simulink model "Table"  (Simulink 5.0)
settings: Solver=FixedStepDiscrete  SolverMode=SingleTasking  StartTime=0.0  StopTime=inf  FixedStep=samplePeriod  RelTol=1e-3  AbsTol=1e-6
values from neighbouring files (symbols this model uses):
  a0 = zeros(1, nAct)    [initialize.m]    (also in quake.m = 0; rspect.m = 1)
  actParamsX = [bulkModulus	* pressCanon,    [initialize.m]
  actParamsY = [bulkModulus	* pressCanon,    [initialize.m]
  actParamsZ = [bulkModulus	* pressCanon,    [initialize.m]
  azMask = zeros(nAcc, 1)    [initialize.m]
  bal = [[ 1  1  1  1  0  0  0  0  0  0  0  0]    [initialize.m]
  cmap = jet    [initialize.m]    (also in tableAnimation.m = self.cmap)
  ea_t = zeros(3, nAcc)    [initialize.m]
  faces = nAct               			+ [ 1  2  3  4    [initialize.m]    (also in tableAnimation.m = self.faces)
  flowCanon = 63090.2    [initialize.m]
  fmax = zeros(nAct, 1)    [initialize.m]
  gasConstant = 1.8    [initialize.m]
  gee = 1.0    (= 1)    [initialize.m]    (also in accelA2T.m = h(24); accelT2A.m = h(24); Test.m)
  inertia = [Ixx 0 0; 0 Iyy 0; 0 0 Izz]    [initialize.m]
  inertiaCanon = 0.1130    (= 0.113)    [initialize.m]
  linAccelCanon = 9800.0    (= 9800)    [initialize.m]    (also in accelA2T.m = h(19); accelT2A.m = h(19); Test.m)
  lines = nAct               			+ [ 1  2  3  4  1    				5  6  7  8  5    				9 10 11 12  9    				0  2  6 10       				0  3  7 11       				0  4  8 12  0];  	lines(find(lines==nAct)) = 0    [initialize.m]    (also in tableAnimation.m = self.lines; viewer.m = 1)
  linVelocCanon = 1000.0    (= 1000)    [initialize.m]    (also in Test.m)
  mass = [massX massY massZ]'    [initialize.m]
  massCanon = 0.4535924e-06    (= 4.535924e-07)    [initialize.m]
  maxDispl = [maxDisplX  			maxDisplY  			maxDisplZ  			maxDisplZ * linVelocCanon / rollRadius  * 180/pi  			maxDisplZ * linVelocCanon / pitchRadius * 180/pi  			min(maxDisplX, maxDisplY) * linVelocCanon / yawRadius * 180/pi]    [initialize.m]
  maxOilVolume = volume * (1 - (precharge/supplyPress)^(1/gasConstant))    (= 32.2704137442)    [initialize.m]
  maxVeloc = [maxVelocX  			maxVelocY  			maxVelocZ  			maxVelocZ * linVelocCanon / rollRadius  * 180/pi  			maxVelocZ * linVelocCanon / pitchRadius * 180/pi  			min(maxVelocX, maxVelocY) * linVelocCanon / yawRadius * 180/pi]    [initialize.m]
  minDispl = -maxDispl    [initialize.m]
  minVeloc = -maxVeloc    [initialize.m]
  nAct = size(rt_t, 2)    [initialize.m]    (also in tableAnimation.m = self.nAct)
  precharge = 2000    [initialize.m]
  pumpFlow = 1e10    (= 10000000000)    [initialize.m]
  ra_t = [  -20.0   -20.0   -92.0 -2590.0  2590.0   -62.0 -2133.0 -2133.0  2133.0  2133.0   -62.0    [initialize.m]    (also in accelA2T.m = [-h9   -h9 -h15 -h10  h10 -h14 -h12 -h12  h12  h12 -h16; accelT2A.m = [-h9   -h9 -h15 -h10  h10 -h14 -h12 -h12  h12  h12 -h16)
  rb_w = [-5692.1 -5692.1  5692.1  5692.1 -2500.0 -2500.0  2500.0  2500.0 -2400.0 -2400.0  2400.0  2400.0    [initialize.m]    (also in tableAnimation.m = rtxrb_w(:,end-nAct+1:end); positT2A.m = [-h4 -h4  h4  h4 -h1 -h1  h1  h1 -h6 -h6  h6  h6)
  returnPress = 50    [initialize.m]
  rgt = -rtg    [initialize.m]
  rotAccelCanon = 1    [initialize.m]    (also in accelA2T.m = h(22); accelT2A.m = h(22); Test.m)
  rotForceCanon = 1000    [initialize.m]    (also in forceA2T.m = h(23); Test.m)
  rotVelocCanon = 1    [initialize.m]    (also in accelA2T.m = h(21); accelT2A.m = h(21); Test.m)
  rt_t = [-3106.4 -3106.4  3106.4  3106.4 -2500.0 -2500.0  2500.0  2500.0 -2400.0 -2400.0  2400.0  2400.0    [initialize.m]    (also in positT2A.m = [rt_tx rt_ty rt_tz])
  rtg = cg    [initialize.m]
  rtx_t = [rt_t	topPlane.topLeft(:)  topPlane.topRight(:)  					topPlane.botRight(:) topPlane.botLeft(:)   					midPlane.topLeft(:)  midPlane.topRight(:)  					midPlane.botRight(:) midPlane.botLeft(:)   					botPlane.topLeft(:)  botPlane.topRight(:)  					botPlane.botRight(:) botPlane.botLeft(:)]    [initialize.m]
  samplePeriod = 1/1024    (= 0.0009765625)    [initialize.m]    (also in viewer.m = eval(getHeaderValue(header, 'DELTA_T')))
  supplyPress = 3000    [initialize.m]
  volume = 160    [initialize.m]    (also in quake.m = volume / 231.0)
  volumeCanon = 3785412.0    (= 3785412)    [initialize.m]
  zlim = [min(rb_w(3,:)) 2*halfLengthZ*lengthCanon]    [initialize.m]
undefined symbols (not defined in the file or in its folder): magnitude
libraries: aerospace x51, simulink x22, simulink_extras x1
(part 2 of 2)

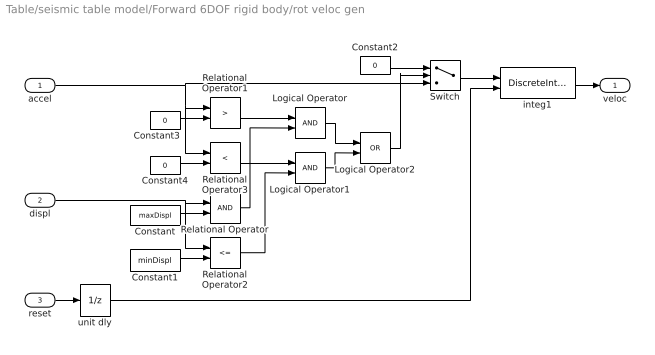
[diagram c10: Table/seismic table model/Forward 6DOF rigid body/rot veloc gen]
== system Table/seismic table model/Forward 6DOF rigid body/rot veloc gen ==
  accel : Inport
  displ : Inport  Port=2
  reset : Inport  Port=3
  Constant : Constant  Value=maxDispl
  Constant1 : Constant  Value=minDispl
  Constant2 : Constant  Value=0
  Constant3 : Constant  Value=0
  Constant4 : Constant  Value=0
  Logical Operator : Logic
  Logical Operator1 : Logic
  Logical Operator2 : Logic  Operator=OR
  Relational Operator : RelationalOperator
  Relational Operator1 : RelationalOperator  Operator=>
  Relational Operator2 : RelationalOperator  Operator=<=
  Relational Operator3 : RelationalOperator  Operator=<
  Switch : Switch  Threshold=0.5
  integ1 : DiscreteIntegrator  ExternalReset=either  LimitOutput=on  UpperSaturationLimit=maxVeloc  LowerSaturationLimit=minVeloc  SampleTime=-1
  unit dly : UnitDelay  SampleTime=-1
  veloc : Outport
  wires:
  reset/1 -> unit dly/1
  displ/1 -> Relational Operator2/1, Relational Operator/1
  Logical Operator1/1 -> Logical Operator2/2
  unit dly/1 -> integ1/2
  Switch/1 -> integ1/1
  Logical Operator2/1 -> Switch/2
  Constant2/1 -> Switch/1
  Logical Operator/1 -> Logical Operator2/1
  Relational Operator3/1 -> Logical Operator1/1
  Constant4/1 -> Relational Operator3/2
  Relational Operator1/1 -> Logical Operator/1
  Constant3/1 -> Relational Operator1/2
  accel/1 -> Switch/3, Relational Operator1/1, Relational Operator3/1
  Constant1/1 -> Relational Operator2/2
  Relational Operator2/1 -> Logical Operator1/2
  Relational Operator/1 -> Logical Operator/2
  Constant/1 -> Relational Operator/2
  integ1/1 -> veloc/1

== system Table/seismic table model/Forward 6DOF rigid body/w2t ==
  rpw : Inport
  11 : Fcn  Expr=cos(u[3])*cos(u[2])-sin(u[3])*sin(u[1])*sin(u[2])
  12 : Fcn  Expr=sin(u[3])*cos(u[2])+cos(u[3])*sin(u[1])*sin(u[2])
  13 : Fcn  Expr=-cos(u[1])*sin(u[2])
  21 : Fcn  Expr=-sin(u[3])*cos(u[1])
  22 : Fcn  Expr=cos(u[3])*cos(u[1])
  23 : Fcn
  31 : Fcn  Expr=cos(u[3])*sin(u[2])+sin(u[3])*sin(u[1])*cos(u[2])
  32 : Fcn  Expr=sin(u[3])*sin(u[2])-cos(u[3])*sin(u[1])*cos(u[2])
  33 : Fcn  Expr=cos(u[1])*cos(u[2])
  9x1->3x3 : simulink/Math Operations/Reshape  OutputDimensionality=Customize  OutputDimensions=[3,3]
  Mux2 : Mux  Orientation=down  Inputs=9
  DCM : Outport
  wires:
  9x1->3x3/1 -> DCM/1
  11/1 -> Mux2/1
  21/1 -> Mux2/2
  31/1 -> Mux2/3
  rpw/1 -> 31/1, 21/1, 11/1, 32/1, 22/1, 12/1, 33/1, 23/1, 13/1
  12/1 -> Mux2/4
  22/1 -> Mux2/5
  32/1 -> Mux2/6
  Mux2/1 -> 9x1->3x3/1
  13/1 -> Mux2/7
  23/1 -> Mux2/8
  33/1 -> Mux2/9

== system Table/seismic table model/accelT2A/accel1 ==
  linacc : Inport
  rotacc : Inport  Port=2
  rotvel : Inport  Port=3
  Sum : Sum  Inputs=+++
  crossprod1 : aerospace/Axes Transformations/3x3 cross product
  crossprod2 : aerospace/Axes Transformations/3x3 cross product
  crossprod3 : aerospace/Axes Transformations/3x3 cross product
  dotprod : simulink/Math Operations/Dot Product
  orient : Constant  Value=ea_t(:,id)
  ra_t : Constant  Value=ra_t(:,id)
  out : Outport
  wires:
  orient/1 -> dotprod/2
  dotprod/1 -> out/1
  linacc/1 -> Sum/1
  Sum/1 -> dotprod/1
  rotacc/1 -> crossprod1/1
  ra_t/1 -> crossprod1/2, crossprod2/2
  crossprod1/1 -> Sum/2
  rotvel/1 -> crossprod2/1, crossprod3/1
  crossprod3/1 -> Sum/3
  crossprod2/1 -> crossprod3/2

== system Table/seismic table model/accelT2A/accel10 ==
  linacc : Inport
  rotacc : Inport  Port=2
  rotvel : Inport  Port=3
  Sum : Sum  Inputs=+++
  crossprod1 : aerospace/Axes Transformations/3x3 cross product
  crossprod2 : aerospace/Axes Transformations/3x3 cross product
  crossprod3 : aerospace/Axes Transformations/3x3 cross product
  dotprod : simulink/Math Operations/Dot Product
  orient : Constant  Value=ea_t(:,id)
  ra_t : Constant  Value=ra_t(:,id)
  out : Outport
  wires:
  crossprod2/1 -> crossprod3/2
  crossprod3/1 -> Sum/3
  rotvel/1 -> crossprod3/1, crossprod2/1
  crossprod1/1 -> Sum/2
  ra_t/1 -> crossprod2/2, crossprod1/2
  rotacc/1 -> crossprod1/1
  Sum/1 -> dotprod/1
  linacc/1 -> Sum/1
  dotprod/1 -> out/1
  orient/1 -> dotprod/2

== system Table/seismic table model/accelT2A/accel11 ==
  linacc : Inport
  rotacc : Inport  Port=2
  rotvel : Inport  Port=3
  Sum : Sum  Inputs=+++
  crossprod1 : aerospace/Axes Transformations/3x3 cross product
  crossprod2 : aerospace/Axes Transformations/3x3 cross product
  crossprod3 : aerospace/Axes Transformations/3x3 cross product
  dotprod : simulink/Math Operations/Dot Product
  orient : Constant  Value=ea_t(:,id)
  ra_t : Constant  Value=ra_t(:,id)
  out : Outport
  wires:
  orient/1 -> dotprod/2
  dotprod/1 -> out/1
  linacc/1 -> Sum/1
  Sum/1 -> dotprod/1
  rotacc/1 -> crossprod1/1
  ra_t/1 -> crossprod1/2, crossprod2/2
  crossprod1/1 -> Sum/2
  rotvel/1 -> crossprod2/1, crossprod3/1
  crossprod3/1 -> Sum/3
  crossprod2/1 -> crossprod3/2

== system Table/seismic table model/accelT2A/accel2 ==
  linacc : Inport
  rotacc : Inport  Port=2
  rotvel : Inport  Port=3
  Sum : Sum  Inputs=+++
  crossprod1 : aerospace/Axes Transformations/3x3 cross product
  crossprod2 : aerospace/Axes Transformations/3x3 cross product
  crossprod3 : aerospace/Axes Transformations/3x3 cross product
  dotprod : simulink/Math Operations/Dot Product
  orient : Constant  Value=ea_t(:,id)
  ra_t : Constant  Value=ra_t(:,id)
  out : Outport
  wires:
  crossprod2/1 -> crossprod3/2
  crossprod3/1 -> Sum/3
  rotvel/1 -> crossprod3/1, crossprod2/1
  crossprod1/1 -> Sum/2
  ra_t/1 -> crossprod2/2, crossprod1/2
  rotacc/1 -> crossprod1/1
  Sum/1 -> dotprod/1
  linacc/1 -> Sum/1
  dotprod/1 -> out/1
  orient/1 -> dotprod/2

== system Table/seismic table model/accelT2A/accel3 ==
  linacc : Inport
  rotacc : Inport  Port=2
  rotvel : Inport  Port=3
  Sum : Sum  Inputs=+++
  crossprod1 : aerospace/Axes Transformations/3x3 cross product
  crossprod2 : aerospace/Axes Transformations/3x3 cross product
  crossprod3 : aerospace/Axes Transformations/3x3 cross product
  dotprod : simulink/Math Operations/Dot Product
  orient : Constant  Value=ea_t(:,id)
  ra_t : Constant  Value=ra_t(:,id)
  out : Outport
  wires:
  orient/1 -> dotprod/2
  dotprod/1 -> out/1
  linacc/1 -> Sum/1
  Sum/1 -> dotprod/1
  rotacc/1 -> crossprod1/1
  ra_t/1 -> crossprod1/2, crossprod2/2
  crossprod1/1 -> Sum/2
  rotvel/1 -> crossprod2/1, crossprod3/1
  crossprod3/1 -> Sum/3
  crossprod2/1 -> crossprod3/2

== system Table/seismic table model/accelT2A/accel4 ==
  linacc : Inport
  rotacc : Inport  Port=2
  rotvel : Inport  Port=3
  Sum : Sum  Inputs=+++
  crossprod1 : aerospace/Axes Transformations/3x3 cross product
  crossprod2 : aerospace/Axes Transformations/3x3 cross product
  crossprod3 : aerospace/Axes Transformations/3x3 cross product
  dotprod : simulink/Math Operations/Dot Product
  orient : Constant  Value=ea_t(:,id)
  ra_t : Constant  Value=ra_t(:,id)
  out : Outport
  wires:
  crossprod2/1 -> crossprod3/2
  crossprod3/1 -> Sum/3
  rotvel/1 -> crossprod3/1, crossprod2/1
  crossprod1/1 -> Sum/2
  ra_t/1 -> crossprod2/2, crossprod1/2
  rotacc/1 -> crossprod1/1
  Sum/1 -> dotprod/1
  linacc/1 -> Sum/1
  dotprod/1 -> out/1
  orient/1 -> dotprod/2

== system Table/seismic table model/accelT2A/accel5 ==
  linacc : Inport
  rotacc : Inport  Port=2
  rotvel : Inport  Port=3
  Sum : Sum  Inputs=+++
  crossprod1 : aerospace/Axes Transformations/3x3 cross product
  crossprod2 : aerospace/Axes Transformations/3x3 cross product
  crossprod3 : aerospace/Axes Transformations/3x3 cross product
  dotprod : simulink/Math Operations/Dot Product
  orient : Constant  Value=ea_t(:,id)
  ra_t : Constant  Value=ra_t(:,id)
  out : Outport
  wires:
  orient/1 -> dotprod/2
  dotprod/1 -> out/1
  linacc/1 -> Sum/1
  Sum/1 -> dotprod/1
  rotacc/1 -> crossprod1/1
  ra_t/1 -> crossprod1/2, crossprod2/2
  crossprod1/1 -> Sum/2
  rotvel/1 -> crossprod2/1, crossprod3/1
  crossprod3/1 -> Sum/3
  crossprod2/1 -> crossprod3/2

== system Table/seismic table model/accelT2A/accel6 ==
  linacc : Inport
  rotacc : Inport  Port=2
  rotvel : Inport  Port=3
  Sum : Sum  Inputs=+++
  crossprod1 : aerospace/Axes Transformations/3x3 cross product
  crossprod2 : aerospace/Axes Transformations/3x3 cross product
  crossprod3 : aerospace/Axes Transformations/3x3 cross product
  dotprod : simulink/Math Operations/Dot Product
  orient : Constant  Value=ea_t(:,id)
  ra_t : Constant  Value=ra_t(:,id)
  out : Outport
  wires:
  crossprod2/1 -> crossprod3/2
  crossprod3/1 -> Sum/3
  rotvel/1 -> crossprod3/1, crossprod2/1
  crossprod1/1 -> Sum/2
  ra_t/1 -> crossprod2/2, crossprod1/2
  rotacc/1 -> crossprod1/1
  Sum/1 -> dotprod/1
  linacc/1 -> Sum/1
  dotprod/1 -> out/1
  orient/1 -> dotprod/2

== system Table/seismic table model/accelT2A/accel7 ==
  linacc : Inport
  rotacc : Inport  Port=2
  rotvel : Inport  Port=3
  Sum : Sum  Inputs=+++
  crossprod1 : aerospace/Axes Transformations/3x3 cross product
  crossprod2 : aerospace/Axes Transformations/3x3 cross product
  crossprod3 : aerospace/Axes Transformations/3x3 cross product
  dotprod : simulink/Math Operations/Dot Product
  orient : Constant  Value=ea_t(:,id)
  ra_t : Constant  Value=ra_t(:,id)
  out : Outport
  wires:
  orient/1 -> dotprod/2
  dotprod/1 -> out/1
  linacc/1 -> Sum/1
  Sum/1 -> dotprod/1
  rotacc/1 -> crossprod1/1
  ra_t/1 -> crossprod1/2, crossprod2/2
  crossprod1/1 -> Sum/2
  rotvel/1 -> crossprod2/1, crossprod3/1
  crossprod3/1 -> Sum/3
  crossprod2/1 -> crossprod3/2

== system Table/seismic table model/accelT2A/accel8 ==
  linacc : Inport
  rotacc : Inport  Port=2
  rotvel : Inport  Port=3
  Sum : Sum  Inputs=+++
  crossprod1 : aerospace/Axes Transformations/3x3 cross product
  crossprod2 : aerospace/Axes Transformations/3x3 cross product
  crossprod3 : aerospace/Axes Transformations/3x3 cross product
  dotprod : simulink/Math Operations/Dot Product
  orient : Constant  Value=ea_t(:,id)
  ra_t : Constant  Value=ra_t(:,id)
  out : Outport
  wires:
  crossprod2/1 -> crossprod3/2
  crossprod3/1 -> Sum/3
  rotvel/1 -> crossprod3/1, crossprod2/1
  crossprod1/1 -> Sum/2
  ra_t/1 -> crossprod2/2, crossprod1/2
  rotacc/1 -> crossprod1/1
  Sum/1 -> dotprod/1
  linacc/1 -> Sum/1
  dotprod/1 -> out/1
  orient/1 -> dotprod/2

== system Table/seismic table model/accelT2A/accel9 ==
  linacc : Inport
  rotacc : Inport  Port=2
  rotvel : Inport  Port=3
  Sum : Sum  Inputs=+++
  crossprod1 : aerospace/Axes Transformations/3x3 cross product
  crossprod2 : aerospace/Axes Transformations/3x3 cross product
  crossprod3 : aerospace/Axes Transformations/3x3 cross product
  dotprod : simulink/Math Operations/Dot Product
  orient : Constant  Value=ea_t(:,id)
  ra_t : Constant  Value=ra_t(:,id)
  out : Outport
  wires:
  orient/1 -> dotprod/2
  dotprod/1 -> out/1
  linacc/1 -> Sum/1
  Sum/1 -> dotprod/1
  rotacc/1 -> crossprod1/1
  ra_t/1 -> crossprod1/2, crossprod2/2
  crossprod1/1 -> Sum/2
  rotvel/1 -> crossprod2/1, crossprod3/1
  crossprod3/1 -> Sum/3
  crossprod2/1 -> crossprod3/2

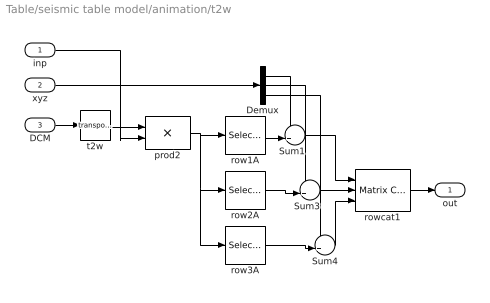
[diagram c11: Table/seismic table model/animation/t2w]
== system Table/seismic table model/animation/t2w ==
  inp : Inport
  xyz : Inport  Port=2
  DCM : Inport  Port=3
  Demux : Demux  Outputs=3
  Sum1 : Sum  Inputs=++|
  Sum3 : Sum  Inputs=++|
  Sum4 : Sum  Inputs=++|
  prod2 : Product  Multiplication=Matrix(*)
  row1A : Selector  InputType=Matrix  Elements=[1 3]  Columns=-1  InputPortWidth=3
  row2A : Selector  InputType=Matrix  Elements=[1 3]  Rows=2  Columns=-1  InputPortWidth=3
  row3A : Selector  InputType=Matrix  Elements=[1 3]  Rows=3  Columns=-1  InputPortWidth=3
  rowcat1 : simulink/Math Operations/Matrix Concatenation  numInports=3  catMethod=Vertical
  t2w : Math  Operator=transpose
  out : Outport
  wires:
  t2w/1 -> prod2/1
  Sum4/1 -> rowcat1/3
  Sum1/1 -> rowcat1/1
  Sum3/1 -> rowcat1/2
  Demux/3 -> Sum4/1
  Demux/2 -> Sum3/1
  row3A/1 -> Sum4/2
  row2A/1 -> Sum3/2
  Demux/1 -> Sum1/1
  prod2/1 -> row2A/1, row3A/1, row1A/1
  DCM/1 -> t2w/1
  inp/1 -> prod2/2
  rowcat1/1 -> out/1
  row1A/1 -> Sum1/2
  xyz/1 -> Demux/1

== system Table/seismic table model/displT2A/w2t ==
  inp : Inport
  xyz : Inport  Port=2
  DCM : Inport  Port=3
  Demux : Demux  Outputs=3
  Sum5 : Sum  Inputs=-+|
  Sum6 : Sum  Inputs=-+|
  Sum7 : Sum  Inputs=-+|
  prod : Product  Multiplication=Matrix(*)
  row1A : Selector  InputType=Matrix  Elements=[1 3]  Columns=-1  InputPortWidth=3
  row2A : Selector  InputType=Matrix  Elements=[1 3]  Rows=2  Columns=-1  InputPortWidth=3
  row3A : Selector  InputType=Matrix  Elements=[1 3]  Rows=3  Columns=-1  InputPortWidth=3
  rowcat : simulink/Math Operations/Matrix Concatenation  numInports=3  catMethod=Vertical
  out : Outport
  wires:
  DCM/1 -> prod/1
  prod/1 -> out/1
  rowcat/1 -> prod/2
  inp/1 -> row3A/1, row2A/1, row1A/1
  xyz/1 -> Demux/1
  row1A/1 -> Sum5/2
  Demux/1 -> Sum5/1
  row2A/1 -> Sum6/2
  row3A/1 -> Sum7/2
  Demux/2 -> Sum6/1
  Demux/3 -> Sum7/1
  Sum6/1 -> rowcat/2
  Sum5/1 -> rowcat/1
  Sum7/1 -> rowcat/3

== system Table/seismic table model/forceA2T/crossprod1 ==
  A : Inport
  B : Inport  Port=2
  colA : Selector  InputType=Matrix  Elements=[1 3]  Rows=-1  Columns=id  InputPortWidth=3
  colB : Selector  InputType=Matrix  Elements=[1 3]  Rows=-1  Columns=id  InputPortWidth=3
  crossprod : aerospace/Axes Transformations/3x3 cross product
  AxB : Outport
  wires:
  colA/1 -> crossprod/1
  colB/1 -> crossprod/2
  A/1 -> colA/1
  B/1 -> colB/1
  crossprod/1 -> AxB/1

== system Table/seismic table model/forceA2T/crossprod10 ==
  A : Inport
  B : Inport  Port=2
  colA : Selector  InputType=Matrix  Elements=[1 3]  Rows=-1  Columns=id  InputPortWidth=3
  colB : Selector  InputType=Matrix  Elements=[1 3]  Rows=-1  Columns=id  InputPortWidth=3
  crossprod : aerospace/Axes Transformations/3x3 cross product
  AxB : Outport
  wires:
  colA/1 -> crossprod/1
  colB/1 -> crossprod/2
  A/1 -> colA/1
  B/1 -> colB/1
  crossprod/1 -> AxB/1

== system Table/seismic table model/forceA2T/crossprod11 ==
  A : Inport
  B : Inport  Port=2
  colA : Selector  InputType=Matrix  Elements=[1 3]  Rows=-1  Columns=id  InputPortWidth=3
  colB : Selector  InputType=Matrix  Elements=[1 3]  Rows=-1  Columns=id  InputPortWidth=3
  crossprod : aerospace/Axes Transformations/3x3 cross product
  AxB : Outport
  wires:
  crossprod/1 -> AxB/1
  B/1 -> colB/1
  A/1 -> colA/1
  colB/1 -> crossprod/2
  colA/1 -> crossprod/1

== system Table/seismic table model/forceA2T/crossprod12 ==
  A : Inport
  B : Inport  Port=2
  colA : Selector  InputType=Matrix  Elements=[1 3]  Rows=-1  Columns=id  InputPortWidth=3
  colB : Selector  InputType=Matrix  Elements=[1 3]  Rows=-1  Columns=id  InputPortWidth=3
  crossprod : aerospace/Axes Transformations/3x3 cross product
  AxB : Outport
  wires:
  colA/1 -> crossprod/1
  colB/1 -> crossprod/2
  A/1 -> colA/1
  B/1 -> colB/1
  crossprod/1 -> AxB/1

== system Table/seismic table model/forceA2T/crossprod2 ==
  A : Inport
  B : Inport  Port=2
  colA : Selector  InputType=Matrix  Elements=[1 3]  Rows=-1  Columns=id  InputPortWidth=3
  colB : Selector  InputType=Matrix  Elements=[1 3]  Rows=-1  Columns=id  InputPortWidth=3
  crossprod : aerospace/Axes Transformations/3x3 cross product
  AxB : Outport
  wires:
  crossprod/1 -> AxB/1
  B/1 -> colB/1
  A/1 -> colA/1
  colB/1 -> crossprod/2
  colA/1 -> crossprod/1

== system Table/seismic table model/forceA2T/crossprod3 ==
  A : Inport
  B : Inport  Port=2
  colA : Selector  InputType=Matrix  Elements=[1 3]  Rows=-1  Columns=id  InputPortWidth=3
  colB : Selector  InputType=Matrix  Elements=[1 3]  Rows=-1  Columns=id  InputPortWidth=3
  crossprod : aerospace/Axes Transformations/3x3 cross product
  AxB : Outport
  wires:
  colA/1 -> crossprod/1
  colB/1 -> crossprod/2
  A/1 -> colA/1
  B/1 -> colB/1
  crossprod/1 -> AxB/1

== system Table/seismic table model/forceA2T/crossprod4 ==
  A : Inport
  B : Inport  Port=2
  colA : Selector  InputType=Matrix  Elements=[1 3]  Rows=-1  Columns=id  InputPortWidth=3
  colB : Selector  InputType=Matrix  Elements=[1 3]  Rows=-1  Columns=id  InputPortWidth=3
  crossprod : aerospace/Axes Transformations/3x3 cross product
  AxB : Outport
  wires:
  crossprod/1 -> AxB/1
  B/1 -> colB/1
  A/1 -> colA/1
  colB/1 -> crossprod/2
  colA/1 -> crossprod/1

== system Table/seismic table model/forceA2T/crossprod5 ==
  A : Inport
  B : Inport  Port=2
  colA : Selector  InputType=Matrix  Elements=[1 3]  Rows=-1  Columns=id  InputPortWidth=3
  colB : Selector  InputType=Matrix  Elements=[1 3]  Rows=-1  Columns=id  InputPortWidth=3
  crossprod : aerospace/Axes Transformations/3x3 cross product
  AxB : Outport
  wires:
  colA/1 -> crossprod/1
  colB/1 -> crossprod/2
  A/1 -> colA/1
  B/1 -> colB/1
  crossprod/1 -> AxB/1

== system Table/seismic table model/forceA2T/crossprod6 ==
  A : Inport
  B : Inport  Port=2
  colA : Selector  InputType=Matrix  Elements=[1 3]  Rows=-1  Columns=id  InputPortWidth=3
  colB : Selector  InputType=Matrix  Elements=[1 3]  Rows=-1  Columns=id  InputPortWidth=3
  crossprod : aerospace/Axes Transformations/3x3 cross product
  AxB : Outport
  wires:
  crossprod/1 -> AxB/1
  B/1 -> colB/1
  A/1 -> colA/1
  colB/1 -> crossprod/2
  colA/1 -> crossprod/1

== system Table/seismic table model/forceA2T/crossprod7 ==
  A : Inport
  B : Inport  Port=2
  colA : Selector  InputType=Matrix  Elements=[1 3]  Rows=-1  Columns=id  InputPortWidth=3
  colB : Selector  InputType=Matrix  Elements=[1 3]  Rows=-1  Columns=id  InputPortWidth=3
  crossprod : aerospace/Axes Transformations/3x3 cross product
  AxB : Outport
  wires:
  colA/1 -> crossprod/1
  colB/1 -> crossprod/2
  A/1 -> colA/1
  B/1 -> colB/1
  crossprod/1 -> AxB/1

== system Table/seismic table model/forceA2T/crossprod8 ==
  A : Inport
  B : Inport  Port=2
  colA : Selector  InputType=Matrix  Elements=[1 3]  Rows=-1  Columns=id  InputPortWidth=3
  colB : Selector  InputType=Matrix  Elements=[1 3]  Rows=-1  Columns=id  InputPortWidth=3
  crossprod : aerospace/Axes Transformations/3x3 cross product
  AxB : Outport
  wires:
  crossprod/1 -> AxB/1
  B/1 -> colB/1
  A/1 -> colA/1
  colB/1 -> crossprod/2
  colA/1 -> crossprod/1

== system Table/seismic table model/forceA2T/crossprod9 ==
  A : Inport
  B : Inport  Port=2
  colA : Selector  InputType=Matrix  Elements=[1 3]  Rows=-1  Columns=id  InputPortWidth=3
  colB : Selector  InputType=Matrix  Elements=[1 3]  Rows=-1  Columns=id  InputPortWidth=3
  crossprod : aerospace/Axes Transformations/3x3 cross product
  AxB : Outport
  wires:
  crossprod/1 -> AxB/1
  B/1 -> colB/1
  A/1 -> colA/1
  colB/1 -> crossprod/2
  colA/1 -> crossprod/1
